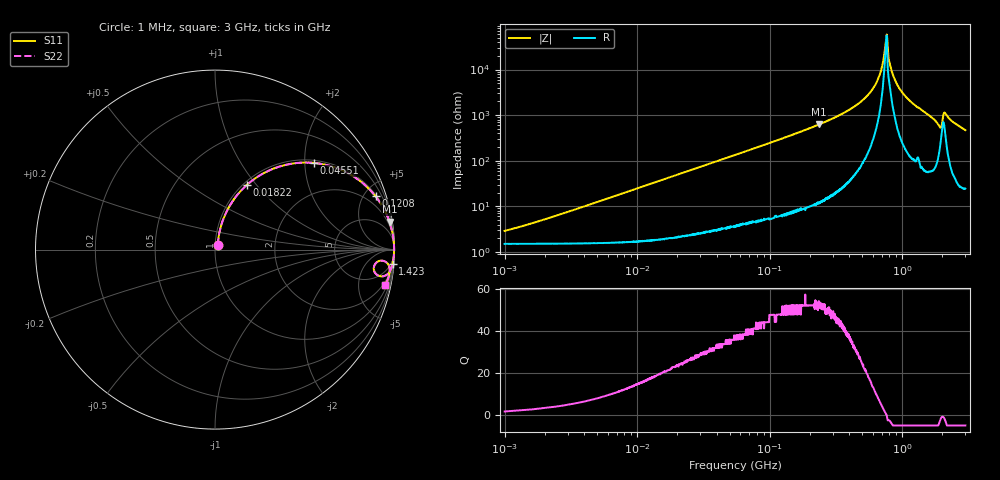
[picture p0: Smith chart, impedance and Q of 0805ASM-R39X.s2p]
!s-Parameter Generated by FASTRON Sdn. Bhd.
!FASTRON P/N : 0805ASM-R39X
!Keysight Technologies: E4991B_MY54100416_A.01.15
!Date: Fri Jun 19 14:52:42 2026
!Version  :Rev00  Fri Jun 19 14:52:42 2026
!Data & Calibration Information:
!Freq  S11  S21  S12  S22
!PortZ  Port1:50+j0  Port2:50+j0
!When reading reference impedance value at option line is always used.
! Remarks : This data is being provided solely for informational purposes.
# Hz S dB R 50
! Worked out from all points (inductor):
!   1601 points, 1 MHz to 3 GHz, reference 50 ohm
!   read as one part in series: L = 395 nH near 1.832 MHz
!   highest Q = 52.5 at 236.1 MHz (marker M1), where L = 423 nH
!   self-resonance near 761.5 MHz
!   S11 on the Smith chart (normalised r, x): 1 MHz: 1.03, +0.05; 18.22 MHz: 1.04, +0.90; 45.51 MHz: 1.07, +2.23; 120.8 MHz: 1.12, +5.97; 1.423 GHz: 2, -25; 3 GHz: 1.48, -9.36
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1000000  -30.90 57.3  -0.13 -1.4  -0.13 -1.4  -30.90 57.3
3804036  -20.60 75.4  -0.17 -5.3  -0.17 -5.3  -20.60 75.4
1.447069e7  -9.60 67.7  -0.66 -19.3  -0.66 -19.3  -9.60 67.7
1.821614e7  -7.89 63.7  -0.94 -23.7  -0.94 -23.7  -7.89 63.7
4.551475e7  -2.69 41.1  -3.63 -47.2  -3.63 -47.2  -2.69 41.1
5.504702e7  -2.02 36.0  -4.61 -52.4  -4.61 -52.4  -2.02 36.0
1.207609e8  -0.52 18.4  -10.00 -70.4  -10.00 -70.4  -0.52 18.4
2.083556e8  -0.18 10.4  -14.80 -78.5  -14.80 -78.5  -0.18 10.4
2.361213e8  -0.14 9.0  -16.10 -79.9  -16.10 -79.9  -0.14 9.0
3.855751e8  -0.05 4.6  -21.90 -83.9  -21.90 -83.9  -0.05 4.6
5.311214e8  -0.02 2.3  -27.90 -85.0  -27.90 -85.0  -0.02 2.3
6.619339e8  -0.02 0.9  -36.20 -81.7  -36.20 -81.7  -0.02 0.9
7.028992e8  -0.02 0.5  -41.00 -76.1  -41.00 -76.1  -0.02 0.5
7.50144e8  -0.02 0.1  -51.70 -37.5  -51.70 -37.5  -0.02 0.1
7.691493e8  -0.01 -0.1  -54.80 42.8  -54.80 42.8  -0.01 -0.1
7.925923e8  -0.02 -0.3  -44.50 67.9  -44.50 67.9  -0.02 -0.3
8.416437e8  -0.02 -0.7  -38.60 77.2  -38.60 77.2  -0.02 -0.7
9.490412e8  -0.02 -1.4  -31.90 83.1  -31.90 83.1  -0.02 -1.4
1.423359e9  -0.06 -4.5  -22.10 82.4  -22.10 82.4  -0.06 -4.5
1.902655e9  -0.49 -9.1  -15.70 65.8  -15.70 65.8  -0.49 -9.1
2.124078e9  -0.28 -4.9  -21.00 66.7  -21.00 66.7  -0.28 -4.9
3e9  -0.28 -11.9  -13.70 75.1  -13.70 75.1  -0.28 -11.9
